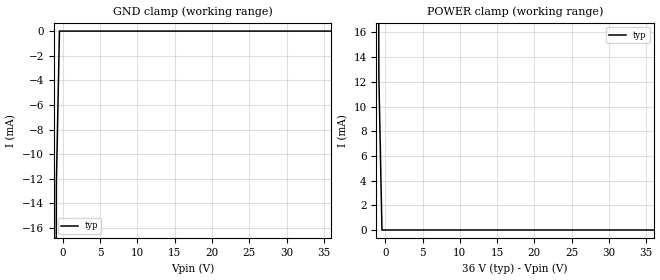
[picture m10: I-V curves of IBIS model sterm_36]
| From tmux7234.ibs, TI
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| sterm_36
[Model]   sterm_36
Model_type   Terminator
|   typ   min   max
C_comp   6.362683e-12   NA   NA
[Voltage Range]   36   NA   NA
[Temperature Range]   27   NA   NA
[Power Clamp Reference]   36   NA   NA
[GND Clamp Reference]   0   NA   NA
[GND Clamp]
|   Voltage   I(typ)   I(min)   I(max)
-5V       -2.15A     NA         NA
-1.273V   -151.4mA   NA         NA
-858.6mV  -12.43mA   NA         NA
-444.4mV  -545.6nA   NA         NA
36V       1.041nA    NA         NA
[POWER Clamp]
|   Voltage   I(typ)   I(min)   I(max)
-5V       2.765A     NA         NA
-1.273V   128.8mA    NA         NA
-858.6mV  12.39mA    NA         NA
-444.4mV  685.3nA    NA         NA
36V       -1.067nA   NA         NA
